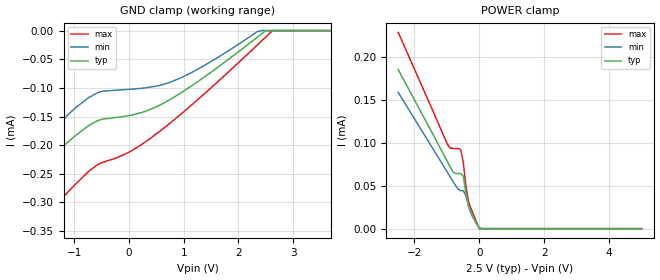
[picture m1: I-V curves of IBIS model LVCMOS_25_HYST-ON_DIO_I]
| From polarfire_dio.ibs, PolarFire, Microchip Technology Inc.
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|   Model LVCMOS_25_HYST-ON_DIO_I
[Model]   LVCMOS_25_HYST-ON_DIO_I
Model_type   Input
Vinl =   0.7
Vinh =   1.7
|   typ   min   max
C_comp   5.210e-12   5.210e-12   5.520e-12
[Model Spec]
Vinh+   1.313   1.247   1.378
Vinh-   1.313   1.247   1.378
Vinl+   1.188   1.128   1.247
Vinl-   1.188   1.128   1.247
[Temperature Range]  25C   100C   -40C
[Voltage Range]  2.5   2.375   2.625
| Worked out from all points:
|   GND clamp passes 1 mA (typ) near -1.92 V on its own axis
[GND Clamp]
| Voltage   I(typ)   I(min)   I(max)
-2.5V     -7.137mA   -7.055mA   -7.618mA
-1.723V   -382.4uA   -596.5uA   -365.8uA
-1.641V   -297.1uA   -416.3uA   -340.2uA
-1.559V   -254.1uA   -303.1uA   -327.5uA
-1.477V   -232.6uA   -235.2uA   -318.2uA
-1.312V   -211.7uA   -173.1uA   -301.2uA
-984.4mV  -183.5uA   -134.9uA   -268.3uA
-574.2mV  -157.1uA   -108.4uA   -233.9uA
546.9mV   -130.8uA   -95.89uA   -176.9uA
2.344V    -11.74uA   -2.033uA   -25.49uA
2.625V    0A         0A         173.1pA
5V        0A         0A         0A
[POWER Clamp]
| Voltage   I(typ)   I(min)   I(max)
-2.5V     185.8uA    159.1uA    229.1uA
-984.4mV  78.33uA    65.88uA    98.56uA
-902.3mV  72.43uA    60.8uA     94.22uA
-820.3mV  66.52uA    55.7uA     93.57uA
-656.2mV  64.34uA    46.12uA    93.57uA
-574.2mV  64.34uA    44.26uA    92.52uA
-492.2mV  61.42uA    44.26uA    76.72uA
-410.2mV  40.87uA    37.93uA    48.28uA
-328.1mV  25.67uA    25.76uA    30.61uA
-246.1mV  18.72uA    16.47uA    22.5uA
0V        0A         1.225uA    0A
5V        0A         0A         0A
